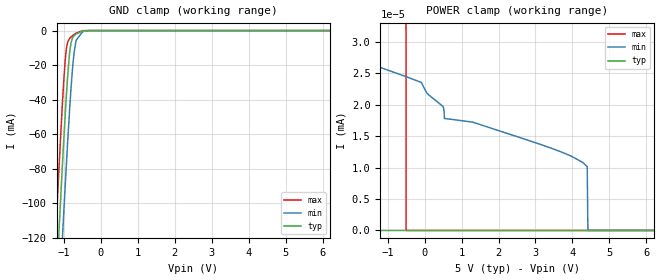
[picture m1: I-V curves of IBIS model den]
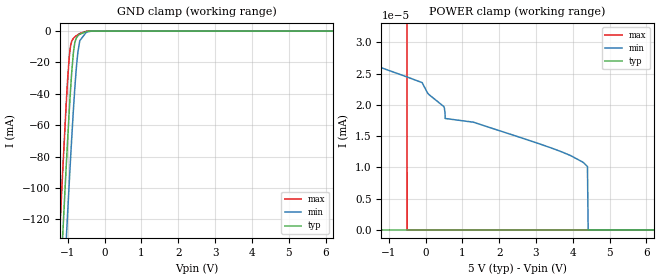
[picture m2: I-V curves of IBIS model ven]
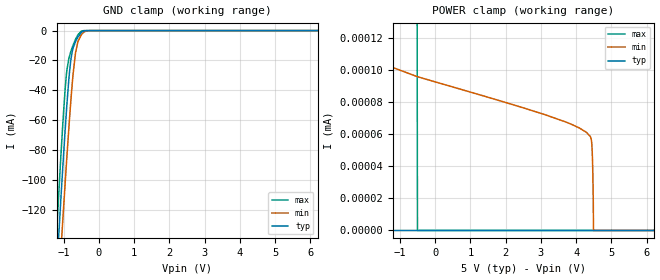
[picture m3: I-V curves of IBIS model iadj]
|Texas Instruments Incorporated
| AUTOMOTIVE USB 2.0 Interface Protection with Short-to-Battery and
| Short-to-Ground Protection, and Adjustable Current Limit
| Marketing part#   Digital Voltage Range   Package-type   #pins
| TPD3S716   4.5V-5.5V   DBQ   16
[IBIS Ver]   4.1
[File name]   tpd3s716.ibs
[File Rev]   1.0
[Date]   02/05/2016
[Source]
| Texas Instruments Incorporated.
| Analog-eLab Design Center, HPA
| 12500 TI Blvd
| Dallas, TX -75243
[Notes]   Revision History:
| Rev 1.0: 02/05/2016
| - Initial version of the model
| - Model generated from simulations in SPECTRE
| - Model matched to SPICE simulation
| - C_comp although listed in numerical order of value are
|   obtained from varying PVT conditions. For PVT conditions for
|   each specific value refer the buffer description under
|   respective [Model]. IBIS model user is responsible for using
|   appropriate C_comp to simulate for Signal Integrity.
[Disclaimer]
| This model is designed as an aid for customers of Texas Instruments.
| TI and its licensors and suppliers make no warranties, either expressed
| or implied, with respect to this  model, including the warranties of
| merchantability or fitness for a particular purpose. The model is
| provided solely on an "as is" basis. The entire risk as to its quality
| and performance is with the customer.
[Copyright]
(C) Copyright 2016 Texas Instruments Incorporated.All rights reserved.
|   TPD3S716
[Component]   TPD3S716
[Manufacturer]   TI
[Package]   |16 DBQ package
|   typ   min   max
R_pkg   0.1   0.08   0.12
L_pkg   1.0nH   0.8nH   1.2nH
C_pkg   0.2pF   0.16pF   0.24pF
[Pin]  signal_name   model_name   R_pin   L_pin   C_pin
1   NC   nc   na   na   na
2   Vbus_con   vbuscon   na   na   na
3   Vbus_con   vbuscon   na   na   na
4   GND   gnd   na   na   na
5   VD-   vdp_vdm   na   na   na
6   VD+   vdp_vdm   na   na   na
7   /VEN   ven   na   na   na
8   /DEN   den   na   na   na
9   Vin   power   na   na   na
10   /FLT   flt   na   na   na
11   D+   dp_dm   na   na   na
12   D-   dp_dm   na   na   na
13   GND   gnd   na   na   na
14   Vbus_sys   nc   na   na   na
15   Vbus_sys   nc   na   na   na
16   Iadj   iadj   na   na   na
| Models and submodels in the file (7): den (Input), ven (Input), iadj (Terminator), flt (I/O_open_drain), dp_dm (Terminator), vdp_vdm (Terminator), vbuscon (Terminator)
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|   den Model
[Model]   den
Model_type   Input
Vinl = 0.8
Vinh = 1.2
|   typ   min   max
|   (nom PVT)   (fast PVT)   (slow PVT)
C_comp   1.505e-12   1.433e-12   1.591e-12
| Where nom  PVT is Nominal Process, 5V, 40C
|   Fast PVT is Strong Process,  5.5V, -40C
|   Slow PVT is Weak Process,   4.5V, 125C
[Voltage Range]   5   4.5   5.5
|Junction Temperature
[Temperature Range]   40   125   -40
[Power Clamp Reference]   5   4.5   5.5
[GND Clamp Reference]   0   0   0
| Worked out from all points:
|   GND clamp passes 1 mA (typ) near -0.57 V on its own axis
|   POWER clamp passes 1 mA (typ) near -3.64 V on its own axis
[GND Clamp]
|   Voltage   I(typ)   I(min)   I(max)
-5V       -1.918A    -1.932A    -1.915A
-1.22V    -153.1mA   -195.4mA   -116.9mA
-1.14V    -118.8mA   -161.3mA   -82.3mA
-1.045V   -79.53mA   -121.9mA   -43.7mA
-1.007V   -64.52mA   -106.4mA   -29.92mA
-945mV    -41.5mA    -82mA      -12.62mA
-895mV    -25.24mA   -63.16mA   -6.529mA
-814.5mV  -8.022mA   -35.58mA   -3.826mA
-725mV    -2.978mA   -12.78mA   -2.269mA
-671mV    -1.989mA   -5.671mA   -1.528mA
-500mV    -345.5uA   -793.6uA   -109uA
10V       0A         0A         0A
[POWER Clamp]
|   Voltage   I(typ)   I(min)   I(max)
-5V       241.8mA    129.1mA    356.3mA
-3.389V   82.02nA    31.02nA    42.56mA
-3.273V   0A         30.61nA    22.09mA
-3.026V   0A         29.8nA     23.95uA
-500mV    0A         24.46nA    0A
-90mV     0A         23.56nA    0A
499mV     0A         19.73nA    0A
535mV     0A         17.83nA    0A
4.297V    0A         10.74nA    0A
4.399V    0A         10.13nA    0A
4.418V    0A         0A         0A
10V       0A         0A         0A
|   ven Model
[Model]   ven
Model_type   Input
Vinl = 0.8
Vinh = 1.2
|   typ   min   max
|   (nom PVT)   (fast PVT)   (slow PVT)
C_comp   1.505e-12   1.433e-12   1.591e-12
| Where nom  PVT is Nominal Process, 5V, 40C
|   Fast PVT is Strong Process,  5.5V, -40C
|   Slow PVT is Weak Process,   4.5V, 125C
[Voltage Range]   5   4.5   5.5
|Junction Temperature
[Temperature Range]   40   125   -40
[Power Clamp Reference]   5   4.5   5.5
[GND Clamp Reference]   0   0   0
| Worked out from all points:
|   GND clamp passes 1 mA (typ) near -0.57 V on its own axis
|   POWER clamp passes 1 mA (typ) near -3.64 V on its own axis
[GND Clamp]
|   Voltage   I(typ)   I(min)   I(max)
-5V       -2.14A     -2.158A    -2.133A
-1.216V   -166.9mA   -214.3mA   -126.4mA
-1.14V    -130.8mA   -178.4mA   -89.95mA
-1.045V   -86.97mA   -134.2mA   -46.99mA
-1.007V   -70.23mA   -117mA     -31.73mA
-945mV    -44.63mA   -89.72mA   -12.87mA
-895mV    -26.68mA   -68.71mA   -6.536mA
-814.5mV  -8.118mA   -38.08mA   -3.826mA
-755mV    -3.84mA    -19.97mA   -2.728mA
-675.5mV  -2.058mA   -6.134mA   -1.586mA
-288.5mV  -2.303uA   -21.65uA   -56.31nA
10V       0A         0A         0A
[POWER Clamp]
|   Voltage   I(typ)   I(min)   I(max)
-5V       241.8mA    129.1mA    356.3mA
-3.389V   82.02nA    31.02nA    42.56mA
-3.273V   0A         30.61nA    22.09mA
-3.026V   0A         29.8nA     23.95uA
-500mV    0A         24.46nA    0A
-90mV     0A         23.56nA    0A
499mV     0A         19.73nA    0A
535mV     0A         17.83nA    0A
4.297V    0A         10.74nA    0A
4.399V    0A         10.13nA    0A
4.418V    0A         0A         0A
10V       0A         0A         0A
|   iadj Model
[Model]   iadj
Model_type   Terminator
|   typ   min   max
|   (nom PVT)   (fast PVT)   (slow PVT)
|   typ   min   max
C_comp   2.386e-12   2.246e-12   2.638e-12
| Where nom  PVT is Nominal Process, 5V, 40C
|   Fast PVT is Strong Process,  5.5V, -40C
|   Slow PVT is Weak Process,   4.5V, 125C
[Voltage Range]   5   4.5   5.5
[Temperature Range]   40   125   -40
[Power Clamp Reference]   5   4.5   5.5
[GND Clamp Reference]   0   0   0
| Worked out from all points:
|   GND clamp passes 1 mA (typ) near -0.48 V on its own axis
|   POWER clamp passes 1 mA (typ) near -3.63 V on its own axis
[GND Clamp]
|   Voltage   I(typ)   I(min)   I(max)
-5V       -1.907A    -1.862A    -1.972A
-1.229V   -174.4mA   -207.4mA   -148.7mA
-1.075V   -112mA     -147.1mA   -83.35mA
-1.024V   -92.03mA   -127.5mA   -63.04mA
-923mV    -55.34mA   -90.51mA   -30.2mA
-803.5mV  -21.49mA   -50.06mA   -14.74mA
-729.5mV  -11.69mA   -28.96mA   -9.745mA
-660.5mV  -7.314mA   -14.79mA   -5.831mA
-594.5mV  -4.356mA   -7.453mA   -2.838mA
-485mV    -1.131mA   -2.449mA   -298.7uA
-225mV    -1.373uA   -20.88uA   -14.46nA
10V       0A         0A         0A
[POWER Clamp]
|   Voltage   I(typ)   I(min)   I(max)
-5V       362.8mA    193.7mA    534.5mA
-3.389V   123.7nA    121.8nA    63.84mA
-3.273V   0A         120.1nA    33.14mA
-3.026V   0A         116.8nA    35.92uA
-500mV    0A         96.07nA    0A
4.297V    0A         61.17nA    0A
4.405V    0A         58.53nA    0A
4.445V    0A         53.48nA    0A
4.473V    0A         35.39nA    0A
4.486V    0A         17.15nA    0A
4.49V     0A         0A         0A
10V       0A         0A         0A
